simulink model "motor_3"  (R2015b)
settings: Solver=FixedStepAuto  StartTime=0.0  StopTime=1  FixedStep=Ts  RelTol=1e-3

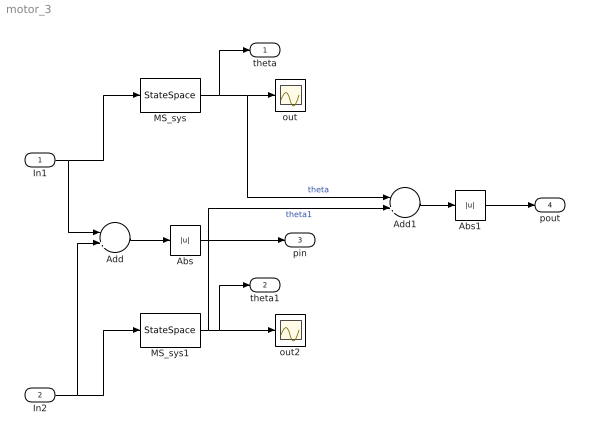
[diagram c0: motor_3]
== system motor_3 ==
  In1 : Inport
  In2 : Inport  Port=2
  Abs : Abs
  Abs1 : Abs
  Add : Sum  Inputs=-+
  Add1 : Sum  Inputs=-+
  MS_sys : StateSpace  A="[ 0  1 ; -5  -2 ]"  B=[ 0 ; 3 ]  C=[ 1 0]  X0=0
  MS_sys1 : StateSpace  A="[ 0  1 ; -5  -2 ];"  B=[ 0 ; 3 ]  C=[1 0]  X0=0
  out : Scope
  out2 : Scope
  theta : Outport
  theta1 : Outport  Port=2
  pin : Outport  Port=3
  pout : Outport  Port=4
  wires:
  MS_sys/1 -> theta/1, Add1/1, out/1  "theta"
  In1/1 -> Add/1, MS_sys/1
  MS_sys1/1 -> Add1/2, theta1/1, out2/1  "theta1"
  In2/1 -> Add/2, MS_sys1/1
  Add/1 -> Abs/1
  Abs/1 -> pin/1
  Add1/1 -> Abs1/1
  Abs1/1 -> pout/1
